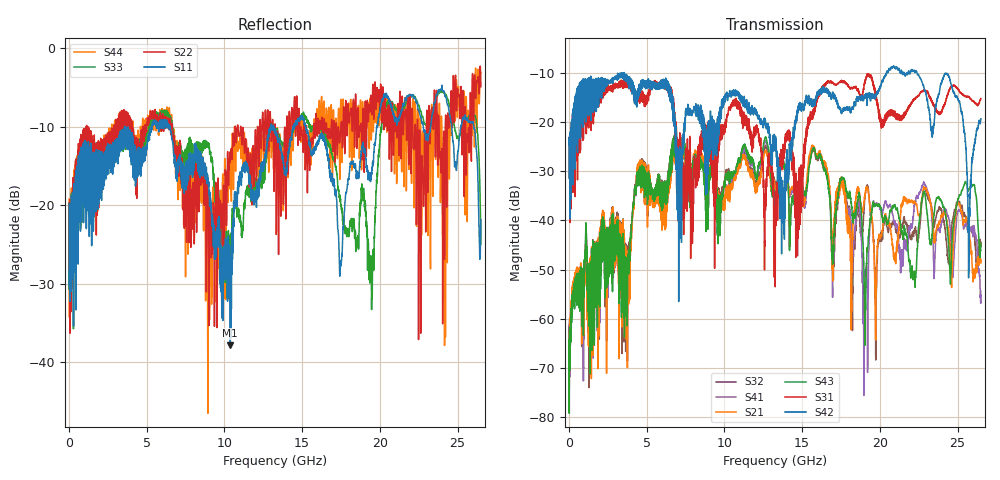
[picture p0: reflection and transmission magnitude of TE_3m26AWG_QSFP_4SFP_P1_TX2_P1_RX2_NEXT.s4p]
!Agilent Technologies,N5222A,MY51421691,A.10.00.00
!Agilent N5222A: A.10.00.00
!Date: Friday, January 30, 2015 12:34:12
!Correction: S11(Full 4 Port(1,2,3,4))
!S12(Full 4 Port(1,2,3,4))
!S13(Full 4 Port(1,2,3,4))
!S14(Full 4 Port(1,2,3,4))
!S21(Full 4 Port(1,2,3,4))
!S22(Full 4 Port(1,2,3,4))
!S23(Full 4 Port(1,2,3,4))
!S24(Full 4 Port(1,2,3,4))
!S31(Full 4 Port(1,2,3,4))
!S32(Full 4 Port(1,2,3,4))
!S33(Full 4 Port(1,2,3,4))
!S34(Full 4 Port(1,2,3,4))
!S41(Full 4 Port(1,2,3,4))
!S42(Full 4 Port(1,2,3,4))
!S43(Full 4 Port(1,2,3,4))
!S44(Full 4 Port(1,2,3,4))
!S4P File: Measurements: <S11,S12,S13,S14>,
!<S21,S22,S23,S24>,
!<S31,S32,S33,S34>,
!<S41,S42,S43,S44>:
# Hz S  dB  R 50.0
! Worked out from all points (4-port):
!   2650 points, 10 MHz to 26.5 GHz, reference 50 ohm
!   strongest paths, dB at 10 MHz, 6.63 GHz, 13.26 GHz, 19.88 GHz, 26.5 GHz:
!     S42: -24.8, -16.1, -25.0, -13.9, -19.4
!     S31: -24.7, -15.5, -42.4, -17.3, -15.3
!     S43: -64.2, -24.7, -35.8, -37.0, -44.7
!     S21: -68.7, -25.3, -33.0, -44.2, -48.6
!     S41: -69.4, -25.1, -36.2, -37.1, -54.4
!     S32: -61.7, -25.0, -32.1, -44.9, -45.3
!   lowest |S11| = -37.9 dB at 10.38 GHz (marker M1), VSWR 1.03, Z = 49 + j0.734 ohm
!   |S11| at or under -10 dB: start of sweep to 3.58 GHz; 6.485 GHz to 12.98 GHz (6.494 GHz wide, 66.7 % of centre); 15.24 GHz to 19.79 GHz (4.55 GHz wide, 26 % of centre)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
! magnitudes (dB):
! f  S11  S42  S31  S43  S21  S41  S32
! 10 MHz  -19.9  -24.8  -24.7  -64.2  -68.7  -69.4  -61.7
! 4.49 GHz  -12.6  -12.8  -13.9  -30.3  -29.1  -30.0  -29.2
! 10.38 GHz  -37.9  -14.5  -17.6  -30.7  -33.9  -33.4  -30.8
! 13.3 GHz  -11.1  -24.7  -36.2  -37.6  -33.6  -37.5  -32.9
! 16.61 GHz  -13.4  -13.9  -12.1  -31.6  -30.4  -31.2  -31.1
! 24.23 GHz  -6.2  -10.2  -15.7  -38.8  -39.0  -37.8  -42.7
! 26.5 GHz  -21.8  -19.4  -15.3  -44.7  -48.6  -54.4  -45.3
